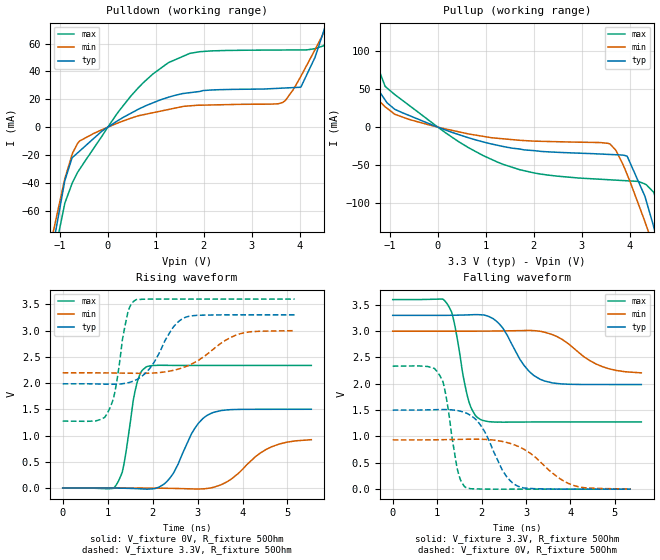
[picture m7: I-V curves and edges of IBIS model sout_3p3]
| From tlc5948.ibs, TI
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|   sout_3p3 Model
[Model]   sout_3p3
Model_type   Output
Polarity   Non-Inverting
Vmeas = 1.65
Vref = 1.65
Cref = 15pF
Rref = 50
|   typ   min   max
|   (nom PVT)   (fast PVT)   (slow PVT)
|C_comp from frequency sweep method (F=8.25MHz)
|C_comp   2.005e-12   1.937e-12   2.064e-12
|ON state : BUFFER OUTPUT TURNED HIGH
|C_comp   2.005e-12   1.937e-12   2.064e-12
|OFF state: BUFFER OUTPUT TURNED LOW
|C_comp   2.244e-12   2.210e-12   2.466e-12
|C_comp from LC tank measurement(L=1nH)
|Resonant Frequency(Hz)   4.510e+09   4.590e+09   4.220e+09
C_comp   1.247e-12   1.204e-12   1.424e-12
|ON state : BUFFER OUTPUT TURNED HIGH
|Resonant Frequency(Hz)   4.510e+09   4.590e+09   4.220e+09
|C_comp   1.247e-12   1.204e-12   1.424e-12
|OFF state: BUFFER OUTPUT TURNED LOW
|Resonant Frequency(Hz)   4.360e+09   4.450e+09   4.130e+09
|C_comp   1.334e-12   1.280e-12   1.487e-12
| Where nom  PVT is Nominal Process, 3.3V, 90C
|   Fast PVT is Strong Process,  3.6V, -40C
|   Slow PVT is Weak Process,   3V, 150C
[Voltage Range]   3.3   3   3.6
|Ambient Temperature   25   85   -40
|Junction Temperature
[Temperature Range]   90   150   -40
[Pullup Reference]   3.3   3   3.6
[Pulldown Reference]   0   0   0
[Power Clamp Reference]   3.3   3   3.6
[GND Clamp Reference]   0   0   0
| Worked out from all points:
|   slope of the pulldown table from 0 to 0.495 V, typ, clamps not added: 48.3 ohm
|   slope of the pullup table from 0 to 0.495 V, typ, clamps not added: 44.7 ohm
|   falling waveform, V_fixture 3.3V, R_fixture 50Ohm: 20-80 % time 562ps typ, 787ps min, 298ps max; typ from 3.3 V to 1.99 V
|   rising waveform, V_fixture 0V, R_fixture 50Ohm: 20-80 % time 517ps typ, 759ps min, 251ps max; typ from 0 V to 1.5 V
|   rising waveform, V_fixture 3.3V, R_fixture 50Ohm: 20-80 % time 530ps typ, 821ps min, 259ps max; typ from 1.99 V to 3.3 V
|   falling waveform, V_fixture 0V, R_fixture 50Ohm: 20-80 % time 527ps typ, 811ps min, 259ps max; typ from 1.5 V to 0 V
[Pulldown]
|   Voltage   I(typ)   I(min)   I(max)
-3.3V     -629.9mA   -494.6mA   -1.043A
-1.084V   -73.93mA   -66.53mA   -86.29mA
-897.6mV  -38.49mA   -37.07mA   -54.73mA
-745.8mV  -22.02mA   -19.68mA   -40.45mA
-588mV    -17.16mA   -9.947mA   -30.22mA
633.6mV   12.83mA    8.142mA    28.2mA
1.706V    24.72mA    15.28mA    52.91mA
3.648V    28.02mA    17.77mA    55.35mA
4.026V    28.92mA    36.66mA    55.43mA
4.583V    78.14mA    73.3mA     64.22mA
4.68V     88.73mA    79.84mA    85.03mA
6.6V      297.9mA    208.9mA    597.4mA
[Pullup]
|   Voltage   I(typ)   I(min)   I(max)
-3.3V     270.7mA    172.6mA    601.6mA
-1.994V   129.8mA    85.33mA    296.7mA
-1.371V   62.52mA    43.68mA    119.6mA
-1.098V   35.75mA    26.81mA    53.72mA
-591mV    15.19mA    10.02mA    28.35mA
1.364V    -25.58mA   -15.41mA   -49.18mA
3.591V    -36.09mA   -22.45mA   -69.53mA
3.947V    -38.45mA   -62.71mA   -70.82mA
4.349V    -98.41mA   -130.7mA   -76.29mA
4.505V    -132.8mA   -158.9mA   -86.74mA
4.759V    -195.2mA   -207.8mA   -173.1mA
6.6V      -668.8mA   -576.9mA   -999.6mA
[Ramp]
R_load = 50
|   typ   min   max
dV/dt_r   0.900487/5.15045e-10   0.560964/7.76766e-10   1.40137/2.50108e-10
dV/dt_f   0.788153/5.6148e-10   0.483054/8.08231e-10   1.39473/2.97402e-10
[Falling Waveform]
V_fixture = 3.3V
V_fixture_min = 3V
V_fixture_max = 3.6V
R_fixture = 50Ohm
|   Time   V(typ)   V(min)   V(max)
0s        3.3V       3V         3.6V
1.21ns    3.301V     3V         3.538V
1.38ns    3.303V     3V         3.179V
1.715ns   3.31V      3V         1.662V
1.97ns    3.312V     3.001V     1.325V
2.405ns   3.131V     3.004V     1.273V
2.955ns   2.351V     3.012V     1.275V
3.33ns    2.082V     2.996V     1.275V
4.73ns    1.987V     2.322V     1.275V
5.595ns   1.986V     2.208V     1.275V
[Rising Waveform]
V_fixture = 0V
V_fixture_min = 0V
V_fixture_max = 0V
R_fixture = 50Ohm
|   Time   V(typ)   V(min)   V(max)
0s        6.899nV    26.38nV    889.5pV
1.185ns   -838.6uV   413.4uV    51.79mV
1.35ns    -3.63mV    493.1uV    402.9mV
1.65ns    -11.87mV   276.2uV    1.994V
1.87ns    -21.62mV   -767.8uV   2.312V
2.39ns    196.1mV    -6.329mV   2.337V
2.935ns   1.134V     -17.98mV   2.335V
3.295ns   1.421V     2.356mV    2.336V
4.655ns   1.5V       788.7mV    2.336V
5.53ns    1.501V     921mV      2.336V
[Rising Waveform]
V_fixture = 3.3V
V_fixture_min = 3V
V_fixture_max = 3.6V
R_fixture = 50Ohm
|   Time   V(typ)   V(min)   V(max)
0s        1.986V     2.195V     1.276V
975ps     1.979V     2.194V     1.398V
1.16ns    1.978V     2.192V     1.83V
1.325ns   1.987V     2.19V      2.811V
1.445ns   2.004V     2.188V     3.331V
1.635ns   2.062V     2.186V     3.59V
1.95ns    2.295V     2.189V     3.6V
2.725ns   3.251V     2.31V      3.6V
3.95ns    3.3V       2.941V     3.6V
5.16ns    3.3V       2.999V     3.6V
[Falling Waveform]
V_fixture = 0V
V_fixture_min = 0V
V_fixture_max = 0V
R_fixture = 50Ohm
|   Time   V(typ)   V(min)   V(max)
0s        1.501V     935mV      2.336V
1.055ns   1.511V     937.9mV    2.164V
1.195ns   1.511V     939.7mV    1.79V
1.455ns   1.493V     943.9mV    378.4mV
1.655ns   1.445V     947.3mV    27.75mV
1.98ns    1.211V     947.6mV    2.317mV
2.46ns    373mV      906.9mV    -432.4uV
2.82ns    54.76mV    813mV      -62.46uV
4.075ns   -78.43uV   68.76mV    10.67uV
5.36ns    25.33uV    1.773mV    5.299uV
